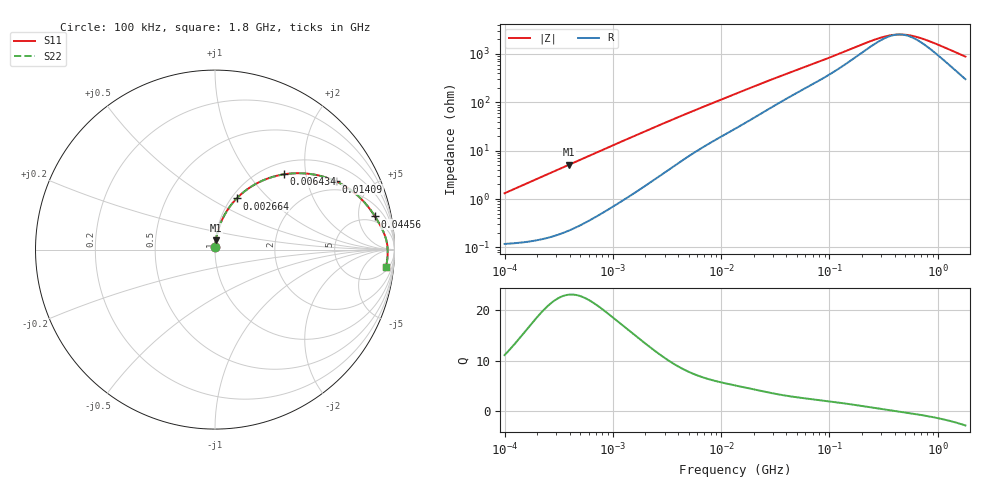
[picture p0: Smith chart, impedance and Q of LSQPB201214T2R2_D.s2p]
! LSQPB201214T2R2_D  S-PARAMETER MODEL  ( General Type )
! Model Generated by TAIYO YUDEN Corporation (http://www.ty-top.com)
! Version 1.0
! TAIYO YUDEN Control No. 100901NG22SB-FKC
! Copyright(c) 2010 TAIYO YUDEN CO.,LTD. All Rights Reserved.
! Product Description (link to TY-COMPAS)
! https://ds.yuden.co.jp/TYCOMPAS/or/detail?pn=LSQPB201214T2R2MD&u=M
! Products Name : Inductors
! Characteristics :
!  Inductance : 2.2 uH , SRF(min) : 350 MHz , DC Resistance(max) : 0.143 Ohm
!  Rated Current : Saturation :1100 mA , Temp Rise : 1000 mA (40 degC)
!  Case Size : 2.0 x 1.25 / 0.079 x 0.049 [mm/inch] , Thickness : 1.4 / 0.056 [mm/inch]
!  (Conditions: Temperature = 25 degC , DC Bias Current/Voltage = 0A / 0V)
! External Node Assignments :
!  1  o---GGG---o  2
! GND o---------o GND
! Frequency Range : 0.1MHz  -  1800MHz  [ 402 STEP ]
# MHz S RI R 50
! Freq[MHz].  S11 Real  S11 Imag  S21 Real  S21 Imag  S12 Real  S12 Imag  S22 Real  S22 Imag
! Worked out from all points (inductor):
!   401 points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, 100 kHz to 1.8 GHz, reference 50 ohm
!   read as one part in series: L = 2.09 uH near 105 kHz
!   highest Q = 23.1 at 394.2 kHz (marker M1), where L = 2.08 uH
!   self-resonance near 437.7 MHz
!   S11 on the Smith chart (normalised r, x): 100 kHz: 1.00, +0.03; 2.664 MHz: 1.06, +0.67; 6.434 MHz: 1.22, +1.51; 14.09 MHz: 1.60, +3.05; 44.56 MHz: 3.72, +8.04; 1.8 GHz: 7, -17
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0.1  0.00135 0.0131  0.9987 -0.0131  0.9987 -0.0131  0.00135 0.0131
0.39422  0.00486 0.0512  0.9951 -0.0512  0.9951 -0.0512  0.00486 0.0512
0.516129  0.00743 0.0666  0.9926 -0.0666  0.9926 -0.0666  0.00743 0.0666
0.863296  0.0178 0.109  0.9822 -0.109  0.9822 -0.109  0.0178 0.109
1.374945  0.0398 0.167  0.9602 -0.167  0.9602 -0.167  0.0398 0.167
1.937403  0.0716 0.2237  0.9284 -0.2237  0.9284 -0.2237  0.0716 0.2237
2.66389  0.1206 0.2847  0.8794 -0.2847  0.8794 -0.2847  0.1206 0.2847
4.039851  0.2229 0.3636  0.7771 -0.3636  0.7771 -0.3636  0.2229 0.3636
6.434145  0.3848 0.4195  0.6152 -0.4195  0.6152 -0.4195  0.3848 0.4195
9.291023  0.5276 0.4218  0.4724 -0.4218  0.4724 -0.4218  0.5276 0.4218
13.41641  0.6599 0.3865  0.3401 -0.3865  0.3401 -0.3865  0.6599 0.3865
14.09005  0.6758 0.3795  0.3242 -0.3795  0.3242 -0.3795  0.6758 0.3795
18.44729  0.7526 0.3348  0.2474 -0.3348  0.2474 -0.3348  0.7526 0.3348
24.15197  0.8113 0.2854  0.1887 -0.2854  0.1887 -0.2854  0.8113 0.2854
44.5561  0.8915 0.1849  0.1085 -0.1849  0.1085 -0.1849  0.8915 0.1849
69.24595  0.9229 0.1309  0.0771 -0.1309  0.0771 -0.1309  0.9229 0.1309
241.5136  0.959 0.0314  0.041 -0.0314  0.041 -0.0314  0.959 0.0314
357.3983  0.9615 0.0103  0.0385 -0.0103  0.0385 -0.0103  0.9615 0.0103
467.921  0.9621 -0.00339  0.0379 0.00339  0.0379 0.00339  0.9621 -0.00339
627.8136  0.9621 -0.0187  0.0379 0.0187  0.0379 0.0187  0.9621 -0.0187
884.6373  0.9612 -0.0388  0.0388 0.0388  0.0388 0.0388  0.9612 -0.0388
1800  0.9529 -0.0976  0.0471 0.0976  0.0471 0.0976  0.9529 -0.0976
